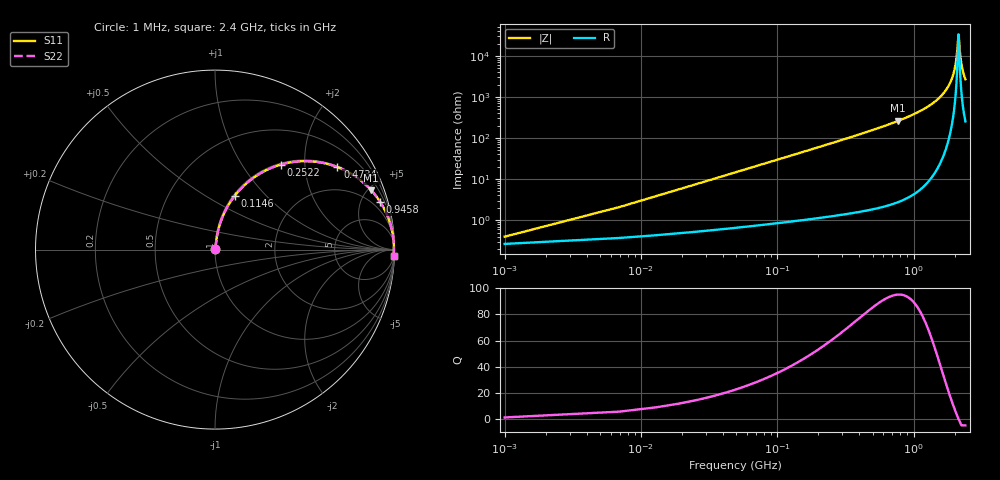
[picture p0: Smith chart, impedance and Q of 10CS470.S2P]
! Coilcraft 1008CS-470 Chip Inductor
! 02 July 2002
# MHZ S MA R 50
!Freq  MagS11  AngS11  MagS21  AngS21  MagS12  AngS12  MagS22  AngS22
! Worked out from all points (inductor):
!   403 points, 1 MHz to 2.4 GHz, reference 50 ohm
!   read as one part in series: L = 47 nH near 12.96 MHz
!   highest Q = 95.2 at 772.4 MHz (marker M1), where L = 54.1 nH
!   self-resonance near 2.136 GHz
!   S11 on the Smith chart (normalised r, x): 1 MHz: 1.01, +0.01; 114.6 MHz: 1.02, +0.68; 252.2 MHz: 1.02, +1.51; 473.4 MHz: 1.04, +2.94; 945.8 MHz: 1.08, +6.95; 2.4 GHz: 6, -54
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1  0.003951 48.0  0.9974 -0.2  0.9974 -0.2  0.003951 48.0
18.94  0.05579 81.9  0.9937 -3.2  0.9937 -3.2  0.05579 81.9
30.9  0.09056 81.3  0.9904 -5.2  0.9904 -5.2  0.09056 81.3
60.8  0.1758 77.7  0.9776 -10.1  0.9776 -10.1  0.1758 77.7
114.62  0.319 69.9  0.9394 -18.6  0.9394 -18.6  0.319 69.9
252.16  0.598 52.3  0.7917 -36.7  0.7917 -36.7  0.598 52.3
401.66  0.771 38.8  0.627 -50.4  0.627 -50.4  0.771 38.8
473.42  0.8223 34.0  0.5593 -55.3  0.5593 -55.3  0.8223 34.0
772.42  0.9312 20.8  0.3549 -68.6  0.3549 -68.6  0.9312 20.8
802.32  0.937 19.9  0.3397 -69.5  0.3397 -69.5  0.937 19.9
945.84  0.9582 16.0  0.2759 -73.4  0.2759 -73.4  0.9582 16.0
1202.98  0.9796 10.9  0.1884 -78.4  0.1884 -78.4  0.9796 10.9
1603.64  0.9934 5.3  0.09169 -83.2  0.09169 -83.2  0.9934 5.3
1848.82  0.9963 2.6  0.04601 -84.1  0.04601 -84.1  0.9963 2.6
2004.3  0.997 1.2  0.0205 -81.0  0.0205 -81.0  0.997 1.2
2070.08  0.9971 0.6  0.0105 -73.4  0.0105 -73.4  0.9971 0.6
2135.86  0.997 0.0  0.002999 -4.1  0.002999 -4.1  0.997 0.0
2147.82  0.997 -0.1  0.003385 27.1  0.003385 27.1  0.997 -0.1
2195.66  0.9969 -0.5  0.009049 69.6  0.009049 69.6  0.9969 -0.5
2237.52  0.9967 -0.8  0.01481 76.9  0.01481 76.9  0.9967 -0.8
2309.28  0.9964 -1.4  0.02467 80.9  0.02467 80.9  0.9964 -1.4
2400  0.9959 -2.1  0.03681 82.5  0.03681 82.5  0.9959 -2.1
